TYPE dut_32Bits :
STRUCT
	
	bBit0	: BIT;
	bBit1	: BIT;
	bBit2	: BIT;
	bBit3	: BIT;
	bBit4	: BIT;
	bBit5	: BIT;
	bBit6	: BIT;
	bBit7	: BIT;
	bBit8	: BIT;
	bBit9	: BIT;
	bBit10	: BIT;
	bBit11	: BIT;
	bBit12	: BIT;
	bBit13	: BIT;
	bBit14	: BIT;
	bBit15	: BIT;
	bBit16	: BIT;
	bBit17	: BIT;
	bBit18	: BIT;
	bBit19	: BIT;
	bBit20	: BIT;
	bBit21	: BIT;
	bBit22	: BIT;
	bBit23	: BIT;
	bBit24	: BIT;
	bBit25	: BIT;
	bBit26	: BIT;
	bBit27	: BIT;
	bBit28	: BIT;
	bBit29	: BIT;
	bBit30	: BIT;
	bBit31	: BIT;
	
END_STRUCT
END_TYPE
